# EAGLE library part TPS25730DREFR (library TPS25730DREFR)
USB Interface IC TPS25730DREFR SARUMAN BG MCM Source: Datasheet
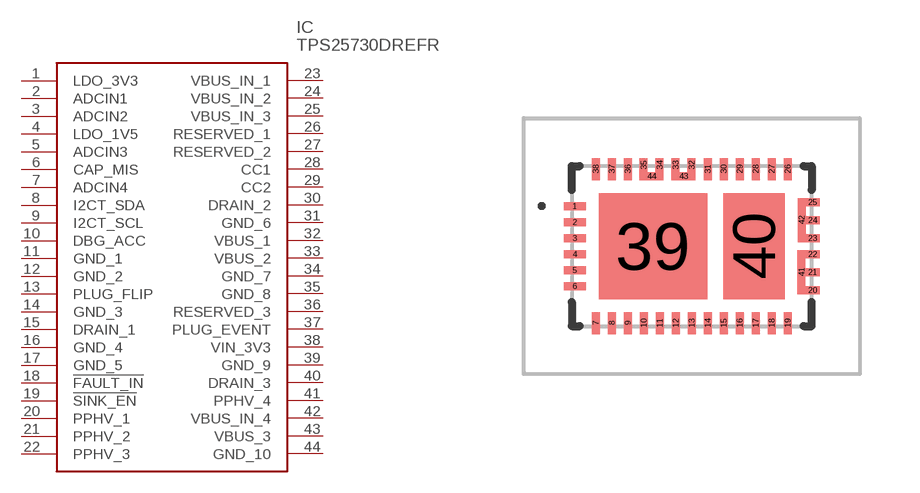
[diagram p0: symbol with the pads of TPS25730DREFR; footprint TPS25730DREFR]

Designator prefix IC

## TPS25730DREFR (Description: USB Interface IC TPS25730DREFR SARUMAN BG MCM; Height: 0.8mm; Manufacturer_Name: Texas Instruments; Manufacturer_Part_Number: TPS25730DREFR; Mouser_Part_Number: 595-TPS25730DREFR; Mouser_Price-Stock: https://www.mouser.co.uk/ProductDetail/Texas-Instruments/TPS25730DREFR?qs=Z%252BL2brAPG1IvmkUK7DRnBA%3D%3D)  [TPS25730DREFR]
1  LDO_3V3
2  ADCIN1
3  ADCIN2
4  LDO_1V5
5  ADCIN3
6  CAP_MIS
7  ADCIN4
8  I2CT_SDA
9  I2CT_SCL
10  DBG_ACC
11  GND_1
12  GND_2
13  PLUG_FLIP
14  GND_3
15  DRAIN_1
16  GND_4
17  GND_5
18  !FAULT_IN
19  !SINK_EN
20  PPHV_1
21  PPHV_2
22  PPHV_3
23  VBUS_IN_1
24  VBUS_IN_2
25  VBUS_IN_3
26  RESERVED_1
27  RESERVED_2
28  CC1
29  CC2
30  DRAIN_2
31  GND_6
32  VBUS_1
33  VBUS_2
34  GND_7
35  GND_8
36  RESERVED_3
37  PLUG_EVENT
38  VIN_3V3
39  GND_9
40  DRAIN_3
41  PPHV_4
42  VBUS_IN_4
43  VBUS_3
44  GND_10

## Footprint TPS25730DREFR (pad centres in mm)
TPS25730DREFR-1
smd 0.55 x 0.2: 1 -2.925,1; 2 -2.925,0.6; 3 -2.925,0.2; 4 -2.925,-0.2; 5 -2.925,-0.6; 6 -2.925,-1
smd 0.2 x 0.55: 7 -2.4,-1.925; 8 -2,-1.925; 9 -1.6,-1.925; 10 -1.2,-1.925; 11 -0.8,-1.925; 12 -0.4,-1.925; 13 0,-1.925; 14 0.4,-1.925; 15 0.8,-1.925; 16 1.2,-1.925; 17 1.6,-1.925; 18 2,-1.925; 19 2.4,-1.925; 26 2.4,1.925; 27 2,1.925; 28 1.6,1.925; 29 1.2,1.925; 30 0.8,1.925; 31 0.4,1.925; 36 -1.6,1.925; 37 -2,1.925; 38 -2.4,1.925
smd 0.35 x 0.2: 20 3.025,-1.1; 21 3.025,-0.65; 22 3.025,-0.2; 23 3.025,0.2; 24 3.025,0.65; 25 3.025,1.1
smd 0.2 x 0.35: 32 -0.001,2.025; 33 -0.401,2.025; 34 -0.801,2.025; 35 -1.201,2.025
smd 2.72 x 2.65: 39 -0.965,0
smd 1.53 x 2.65: 40 1.56,0
smd 0.2 x 1.1: 41 2.749,-0.65; 42 2.75,0.65
smd 0.6 x 0.2: 43 -0.201,1.75; 44 -1.001,1.75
